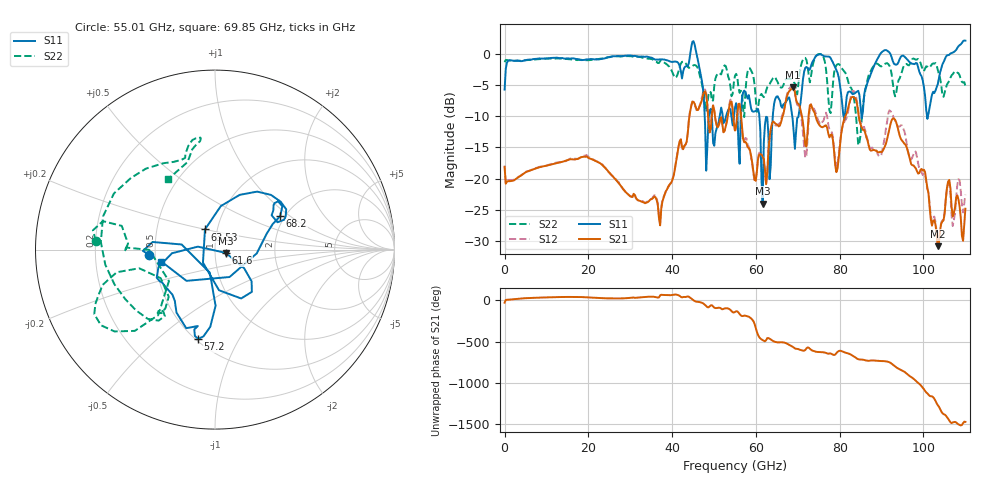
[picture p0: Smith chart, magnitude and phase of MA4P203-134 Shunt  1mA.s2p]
!Keysight Technologies,N5247B,US61255204,A.15.70.20
!Date: Friday, October 21, 2022 15:20:11
!Correction: S11(C  4-Port  )
!S31(C  4-Port  )
!S13(C  4-Port  )
!S33(C  4-Port  )
!S2P File: Measurements: S11, S31, S13, S33:
# Hz S  dB  R 50
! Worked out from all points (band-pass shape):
!   401 points, 10 MHz to 110 GHz, reference 50 ohm
!   highest |S21| = -5.38 dB at 68.75 GHz (marker M1); lowest = -30.8 dB at 103.4 GHz (marker M2)
!   |S21| within 3 dB of the highest: 66.93 GHz to 70.42 GHz (3.493 GHz wide, 5.09 % of centre); 82.13 GHz to 84.2 GHz (2.072 GHz wide, 2.49 % of centre)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
!   lowest |S11| = -24.0 dB at 61.6 GHz (marker M3), VSWR 1.13, Z = 56.4 - j2.09 ohm
!   |S11| at or under -10 dB: 49.45 GHz to 51.37 GHz (1.914 GHz wide, 3.8 % of centre); 60.82 GHz to 64.03 GHz (3.213 GHz wide, 5.15 % of centre); 68.67 GHz to 70.16 GHz (1.497 GHz wide, 2.16 % of centre)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
!   |S22| runs from -14.7 to -0.1 dB; largest |S21 - S12| = 0.17
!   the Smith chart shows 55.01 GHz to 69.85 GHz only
!   S11 on the Smith chart (normalised r, x): 55.01 GHz: 0.46, -0.03; 57.2 GHz: 0.52, -0.69; 61.6 GHz: 1.13, -0.04; 63.53 GHz: 0.87, +0.20; 68.2 GHz: 1.89, +0.85; 69.85 GHz: 0.54, -0.08
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1e7  -5.75 -174.7  -18.14 -29.9  -17.90 -30.0  -1.36 -174.9
1.843332e10  -1.03 145.8  -16.54 37.8  -16.52 37.6  -1.00 145.4
3.685665e10  -0.95 154.6  -26.30 33.7  -25.96 33.9  -1.50 154.3
4.51059e10  1.99 85.4  -7.70 -1.2  -7.66 -3.4  -1.85 115.6
4.813062e10  -18.73 59.1  -6.57 -71.3  -6.40 -71.9  -9.28 113.3
5.5005e10  -8.65 -175.7  -12.31 -142.5  -12.56 -144.2  -3.54 175.9
5.72048e10  -5.92 -100.7  -14.18 173.9  -14.04 -177.7  -10.15 -145.6
6.16044e10  -23.99 -17.0  -16.51 -122.7  -16.60 -120.9  -6.76 -132.8
6.352922e10  -18.02 116.4  -12.07 -113.7  -12.42 -110.9  -4.54 -161.0
6.82038e10  -7.78 27.2  -5.84 173.4  -5.38 170.1  -4.02 97.5
6.875375e10  -10.43 17.0  -5.38 157.9  -5.10 153.8  -4.30 97.9
6.985365e10  -10.30 -167.4  -7.92 131.5  -8.19 130.9  -6.53 123.6
7.342832e10  -1.41 178.4  -8.70 112.3  -8.68 107.5  -2.27 156.4
7.645305e10  -0.45 -165.5  -11.54 87.2  -9.94 118.8  -1.30 148.2
7.947778e10  -3.04 -147.6  -18.42 95.7  -17.61 94.2  -1.70 -137.1
8.415235e10  -6.07 -38.8  -8.16 13.2  -7.70 18.0  -12.30 -169.6
8.745205e10  -3.20 49.8  -15.54 -8.6  -15.17 4.9  -2.71 53.6
9.185165e10  0.21 88.7  -12.04 -30.1  -9.07 -22.8  -1.92 76.1
9.817608e10  -1.50 176.0  -18.38 105.0  -15.72 103.8  -0.97 -174.4
1.034006e11  -4.90 -37.7  -30.81 171.3  -30.81 174.9  -2.59 -110.5
1.069753e11  0.16 10.5  -26.04 -36.1  -27.58 -39.5  -3.29 -23.5
1.1e11  2.08 46.2  -24.81 -30.1  -22.58 -28.6  -5.17 10.2
